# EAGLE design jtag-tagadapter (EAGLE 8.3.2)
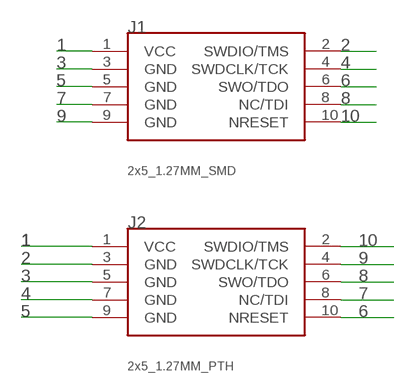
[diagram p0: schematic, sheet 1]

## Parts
J1  ARM_10SMD  [2X5_1.27MM_SMD]
J2  ARM_10PTH  [2X5_1.27MM_PTH]

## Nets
1: J1.1(VCC) J2.1(VCC)
2: J1.2(SWDIO/TMS) J2.3(GND)
3: J1.3(GND) J2.5(GND)
4: J1.4(SWDCLK/TCK) J2.7(GND)
5: J1.5(GND) J2.9(GND)
6: J1.6(SWO/TDO) J2.10(NRESET)
7: J1.7(GND) J2.8(NC/TDI)
8: J1.8(NC/TDI) J2.6(SWO/TDO)
9: J1.9(GND) J2.4(SWDCLK/TCK)
10: J1.10(NRESET) J2.2(SWDIO/TMS)

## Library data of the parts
J1 = fab:ARM_10; PACKAGE: 2x5_1.27MM_SMD
J2 = fab:ARM_10; PACKAGE: 2x5_1.27MM_PTH

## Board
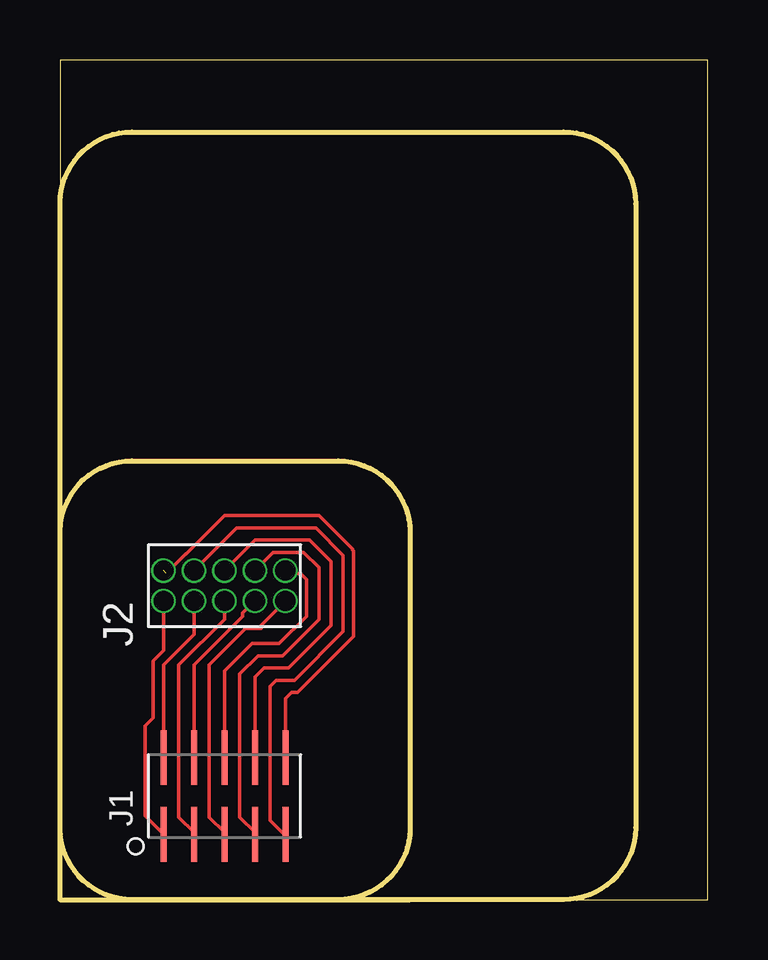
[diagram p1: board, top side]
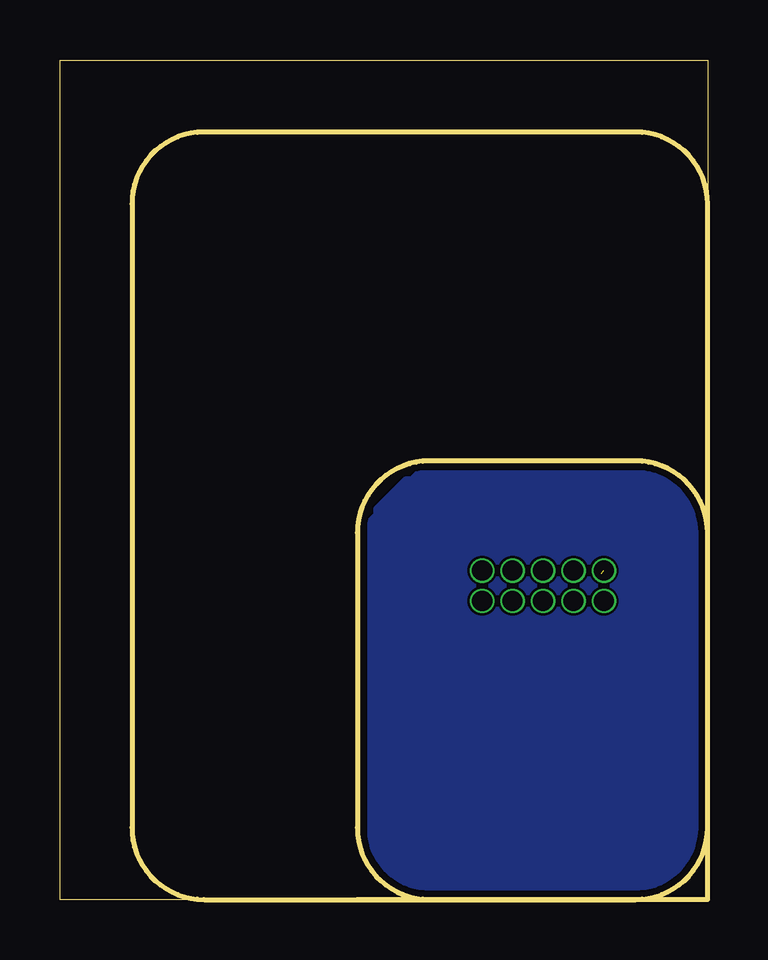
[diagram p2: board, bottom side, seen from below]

Size 27 x 35 mm. Coordinates in mm from the lower left corner, seen from the top.
Outline: 0,3 0,0 3,0
Outline: 0,3 0,15.28
Outline: 0,15.28 0,18.28 0,35 27,35 27,0 14.6,0 11.6,0
Outline: 3,0 11.6,0
Outline: 0,15.28 arc-90 3,18.28 11.6,18.28 arc-90 14.6,15.28 14.6,3 arc-90 11.6,0
Outline: 3,0 arc-90 0,3
Copper layers (1*16): Top 0.035mm / dielectric 1.5mm / Bottom 0.035mm
Design rules "default *": minimum track width 7mil, minimum drill 0.35mm, track to track 4mil, track to pad 4mil, pad to pad 4mil, via to via 4mil, smd to smd 4mil, copper to edge 11mil, drill to drill 11mil, minimum pad ring 3mil, minimum via ring 8mil, stop-mask expansion 4mil, vias tented up to drill 0mil, thermal gap 10mil
Milling: 8 lines

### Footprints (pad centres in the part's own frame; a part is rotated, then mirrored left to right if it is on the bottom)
2X5_1.27MM_SMD = smd 2.286 x 0.254: 1 -1.6,2.54; 2 1.6,2.54; 3 -1.6,1.27; 4 1.6,1.27; 5 -1.6,0; 6 1.6,0; 7 -1.6,-1.27; 8 1.6,-1.27; 9 -1.6,-2.54; 10 1.6,-2.54
2X5_1.27MM_PTH = drill 0.838 pad 1.016: 1 -0.635,2.54; 2 0.635,2.54; 3 -0.635,1.27; 4 0.635,1.27; 5 -0.635,0; 6 0.635,0; 7 -0.635,-1.27; 8 0.635,-1.27; 9 -0.635,-2.54; 10 0.635,-2.54

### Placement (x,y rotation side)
J1  6.86,4.32 90 top
J2  6.86,13.08 90 top

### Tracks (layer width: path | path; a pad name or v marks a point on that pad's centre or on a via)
1
  Top 0.152: J1.1 3.56,3.48 3.56,7.24 3.89,7.57 3.89,9.96 4.32,10.39 J2.1
2
  Top 0.152: J1.2 4.32,9.78 5.59,11.05 J2.3
3
  Top 0.152: J1.3 5.59,2.79 4.95,3.43 4.95,9.78 6.86,11.68 J2.5
4
  Top 0.152: J1.4 5.59,9.78 7.62,11.81 7.62,11.94 J2.7
5
  Top 0.152: J1.5 6.86,2.79 6.22,3.43 6.22,9.78 7.75,11.3 8.38,11.3 8.38,11.43 J2.9
6
  Top 0.152: J1.6 6.86,9.53 8,10.67 9.14,10.67 10.29,11.81 10.29,13.34 10.03,13.59 9.53,13.59 J2.10
7
  Top 0.152: J1.7 8.13,2.79 7.49,3.43 7.49,9.4 8.26,10.16 9.27,10.16 10.79,11.68 10.79,13.84 10.16,14.48 9.14,14.48 | 9.14,14.48 9.02,14.48 | 9.14,14.48 8.89,14.48 J2.8
8
  Top 0.152: J1.8 8.13,9.27 8.51,9.65 9.53,9.65 11.3,11.43 11.3,14.1 10.41,14.99 8.13,14.99 J2.6
9
  Top 0.152: J1.9 9.35,2.72 8.76,3.3 8.76,8.89 9.02,9.14 9.78,9.14 11.81,11.18 11.81,14.35 10.67,15.49 7.37,15.49 J2.4
10  (1 unrouted)
  Top 0.152: 4.42,13.59 5.25,14.41 5.27,14.41 6.86,16 10.79,16 12.19,14.61 12.19,14.58 12.24,14.53 12.24,10.97 9.91,8.64 9.65,8.64 9.4,8.38 J1.10
N$3
  pour Bottom (rank 2): 12.09,0 2,0 1.75,0.25 1.5,0.25 0.25,1.5 0.25,1.75 0,2 0,15.78 0.25,16.03 0.25,16.28 1.5,17.53 1.75,17.53 2,17.78 12.09,17.78 12.34,17.53 12.59,17.53 13.84,16.28 13.84,16.03 14.09,15.78 14.09,2 13.84,1.75 13.84,1.25 13.09,0.5 12.84,0.5 12.59,0.25 12.34,0.25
